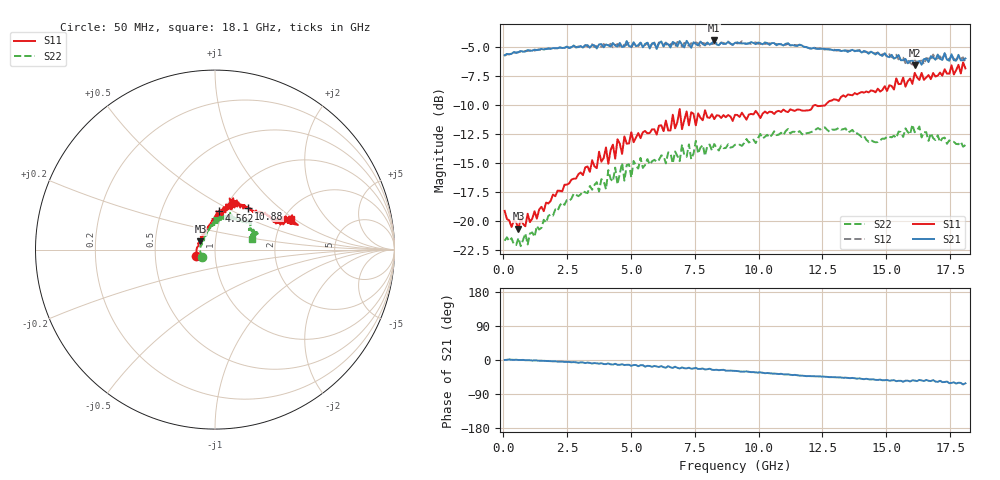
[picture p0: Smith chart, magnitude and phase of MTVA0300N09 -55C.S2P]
! Network Analyzer HP8720D.06.14 Serial No. US36140669
! 28 Jun 2005  09:13:43
! Frequency  S11  S21  S12  S22
# HZ  S  DB R 50
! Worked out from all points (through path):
!   201 points, 50 MHz to 18.1 GHz, reference 50 ohm
!   highest |S21| = -4.45 dB at 8.263 GHz (marker M1); lowest = -6.6 dB at 16.11 GHz (marker M2)
!   group delay of S21, straight-line fit = 10.3 ps
!   lowest |S11| = -20.7 dB at 591.5 MHz (marker M3), VSWR 1.20, Z = 42.3 + j3.86 ohm
!   |S11| at or under -10 dB: start of sweep to 12.62 GHz
!   |S22| runs from -22.2 to -11.7 dB; largest |S21 - S12| = 0.037
!   S11 on the Smith chart (normalised r, x): 50 MHz: 0.81, -0.05; 4.562 GHz: 0.95, +0.43; 10.88 GHz: 1.27, +0.64; 18.1 GHz: 2.19, +0.93
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5e7  -19.12 -162.5  -5.72 0.0  -5.76 0.2  -21.69 -148.1
5.915e8  -20.66 150.8  -5.47 0.0  -5.44 0.1  -21.45 154.6
9.525e8  -19.37 137.5  -5.28 -0.5  -5.35 -0.3  -22.02 139.8
3.1185e9  -16.04 93.9  -5.06 -6.6  -5.06 -7.1  -17.43 101.3
4.5625e9  -13.34 84.6  -4.66 -12.6  -4.95 -12.5  -15.92 83.0
6.09675e9  -11.79 71.4  -4.69 -18.5  -4.62 -17.9  -14.73 75.8
6.548e9  -12.20 67.2  -5.05 -19.2  -4.78 -21.0  -14.16 75.0
6.63825e9  -10.84 70.6  -4.57 -21.0  -4.68 -18.8  -15.03 70.5
6.7285e9  -12.02 75.2  -4.70 -17.7  -5.02 -19.0  -14.01 67.9
6.909e9  -10.36 70.6  -4.50 -22.3  -4.65 -20.0  -14.84 67.0
6.99925e9  -12.09 71.0  -4.83 -19.6  -4.99 -22.2  -13.41 67.1
7.17975e9  -10.56 74.1  -4.48 -22.0  -4.83 -20.4  -14.46 61.8
7.27e9  -11.76 69.4  -4.78 -20.4  -4.90 -23.0  -13.39 65.7
7.36025e9  -10.64 63.2  -5.07 -23.0  -4.68 -21.7  -14.67 69.9
7.54075e9  -11.75 65.1  -4.75 -20.7  -4.62 -24.2  -13.09 67.8
8.26275e9  -11.22 66.3  -4.45 -26.3  -4.72 -27.0  -13.37 55.1
9.075e9  -10.85 62.1  -4.65 -28.8  -4.62 -29.0  -13.43 51.5
1.088e10  -10.61 51.0  -4.78 -36.4  -4.75 -37.2  -12.39 42.4
1.21435e10  -10.05 43.5  -5.10 -42.6  -5.05 -42.7  -12.28 42.9
1.512175e10  -8.30 23.1  -5.89 -54.7  -5.64 -54.4  -12.75 27.6
1.61145e10  -7.24 22.5  -6.58 -54.3  -6.08 -54.8  -12.35 24.2
1.81e10  -6.85 21.7  -6.00 -61.5  -6.30 -62.0  -13.46 16.8
